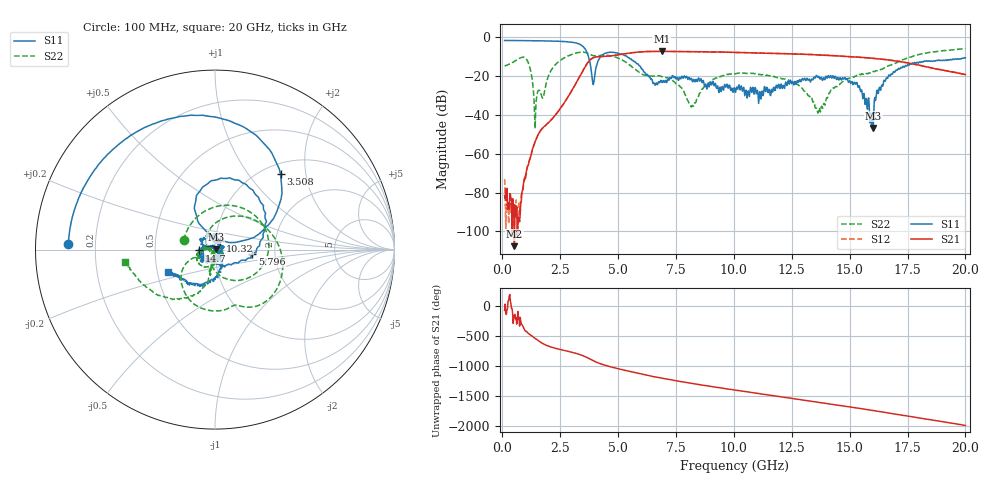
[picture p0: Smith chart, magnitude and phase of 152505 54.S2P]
!  2-Port S-parameters saved by WinCal
! VAR MeasName=S-Parameters (CALIBRATED_DATA) read from VNA (N5230C)
! VAR MeasDate=4/10/2015 9:34:04 AM
! VAR NAME=152505 54
! VAR FILENAME=152505 54.S2P
! VAR DATE=4/10/2015 9:34:04 AM
! VAR PHYS_PORTS=1,2
# Hz S DB R 50
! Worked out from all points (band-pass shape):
!   801 points, 100 MHz to 20 GHz, reference 50 ohm
!   highest |S21| = -7.34 dB at 6.891 GHz (marker M1); lowest = -107.6 dB at 522.9 MHz (marker M2)
!   |S21| within 3 dB of the highest: 4.004 GHz to 15.37 GHz (11.37 GHz wide, 117 % of centre); 15.39073 GHz to 15.40312 GHz (12.39 MHz wide, 0.0805 % of centre)
!   lowest |S11| = -46.8 dB at 16.02 GHz (marker M3), VSWR 1.01, Z = 50.4 + j0.151 ohm
!   |S11| at or under -10 dB: 3.72 GHz to 4.249 GHz (528.9 MHz wide, 13.3 % of centre); 5.379 GHz to end of sweep
!   |S22| runs from -47.0 to -5.9 dB; largest |S21 - S12| = 0.0057
!   S11 on the Smith chart (normalised r, x): 100 MHz: 0.10, +0.02; 3.508 GHz: 1.19, +1.45; 5.796 GHz: 1.52, -0.07; 10.32 GHz: 1.05, +0.10; 14.7 GHz: 0.83, -0.01; 20 GHz: 0.57, -0.16
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1e8  -1.75 177.6  -81.58 -67.8  -73.20 -61.0  -14.84 163.0
5.22875e8  -1.77 167.5  -107.59 -142.2  -99.88 -146.7  -12.49 90.6
1.070125e9  -1.84 154.4  -67.14 -68.0  -68.12 -63.7  -11.85 -34.8
1.468125e9  -1.90 144.1  -52.26 172.7  -52.36 172.2  -32.38 28.2
2.289e9  -2.11 119.7  -40.22 22.2  -40.17 22.0  -14.27 68.9
3.43325e9  -4.33 57.1  -18.23 -94.2  -18.27 -94.0  -7.77 -34.8
3.507875e9  -5.09 49.0  -16.66 -105.5  -16.68 -105.5  -7.79 -41.5
3.93075e9  -24.48 75.5  -10.63 174.5  -10.66 174.5  -9.55 -68.3
4.502875e9  -8.19 88.2  -9.87 92.1  -9.93 92.2  -9.37 -95.1
5.796375e9  -13.62 -6.3  -7.81 -29.5  -7.82 -29.3  -17.13 -158.2
6.741625e9  -23.09 -150.8  -7.35 -105.7  -7.34 -105.9  -19.89 -154.0
6.890875e9  -23.37 -162.9  -7.34 -116.7  -7.36 -116.6  -20.39 -156.8
8.184375e9  -21.76 109.5  -7.49 157.3  -7.52 157.2  -35.60 -136.2
1.005e10  -27.94 75.9  -7.86 45.7  -7.91 45.7  -18.93 -127.0
1.032362e10  -25.14 61.1  -7.98 30.2  -7.96 30.4  -18.44 -136.9
1.201512e10  -24.93 -86.5  -8.54 -64.4  -8.48 -64.2  -21.17 -177.2
1.338325e10  -21.76 -135.5  -9.06 -141.1  -9.00 -141.0  -32.10 175.9
1.37315e10  -21.65 -141.8  -9.24 -161.0  -9.22 -160.9  -38.61 -105.9
1.470162e10  -20.90 -177.0  -9.89 143.8  -9.85 143.0  -22.90 -91.6
1.602e10  -46.83 19.2  -10.95 66.1  -10.95 66.2  -17.76 -103.8
1.669162e10  -19.54 -67.5  -11.81 24.8  -11.81 24.6  -14.72 -102.0
2e10  -10.69 -154.2  -19.33 177.1  -19.33 177.4  -5.91 -172.1
